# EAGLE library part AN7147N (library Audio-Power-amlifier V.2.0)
The AN7147N is an integrated circuit designed for power amplifier of 5.3W (12.0V, 3½) output. Stereo operation is enabled due to incorporating two amps. on one chip. It makes high reliability by smaller quiescent current compared with power amp. current and protectors built in. As quiescent circuit current is very small, it is most suitably used for battery operated set such as radio cassette recorder. Furthermore, low distortion and low noise are realized and external components are very few. 12-pin SIL package enabled compact and high integrated set
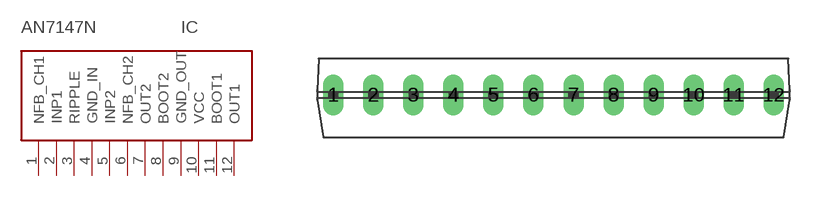
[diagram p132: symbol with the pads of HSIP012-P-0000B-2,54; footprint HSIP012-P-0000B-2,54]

Designator prefix IC

## AN7147N  [HSIP012-P-0000B-2,54]
1  NFB_CH1
2  INP1  in
3  RIPPLE
4  GND_IN  pwr
5  INP2  in
6  NFB_CH2
7  OUT2  out
8  BOOT2
9  GND_OUT  pwr
10  VCC  pwr
11  BOOT1
12  OUT1  out

## Footprint HSIP012-P-0000B-2,54 (pad centres in mm)
drill 0.8 long: 1 -13.97,0; 2 -11.43,0; 3 -8.89,0; 4 -6.35,0; 5 -3.81,0; 6 -1.27,0; 7 1.27,0; 8 3.81,0; 9 6.35,0; 10 8.89,0; 11 11.43,0; 12 13.97,0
